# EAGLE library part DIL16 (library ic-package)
Dual In Line / Socket
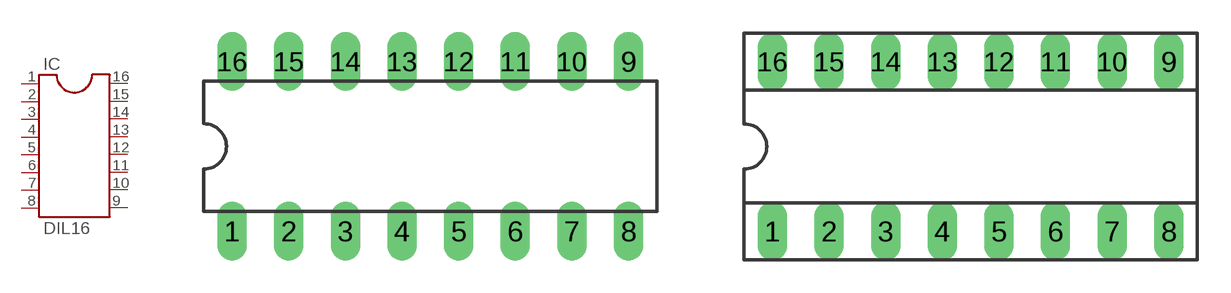
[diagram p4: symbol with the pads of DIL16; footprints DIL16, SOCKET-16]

Designator prefix IC

## DIL16  [DIL16]
1  1  pas
2  2  pas
3  3  pas
4  4  pas
5  5  pas
6  6  pas
7  7  pas
8  8  pas
9  9  pas
10  10  pas
11  11  pas
12  12  pas
13  13  pas
14  14  pas
15  15  pas
16  16  pas

## DIL16S  [SOCKET-16]
Pads as for DIL16

## Footprint DIL16 (pad centres in mm)
Dual In Line Package
drill 0.813 long: 1 -8.89,-3.81; 2 -6.35,-3.81; 3 -3.81,-3.81; 4 -1.27,-3.81; 5 1.27,-3.81; 6 3.81,-3.81; 7 6.35,-3.81; 8 8.89,-3.81; 9 8.89,3.81; 10 6.35,3.81; 11 3.81,3.81; 12 1.27,3.81; 13 -1.27,3.81; 14 -3.81,3.81; 15 -6.35,3.81; 16 -8.89,3.81

## Footprint SOCKET-16 (pad centres in mm)
Dual In Line Socket
drill 0.813 long: 1 -8.89,-3.81; 2 -6.35,-3.81; 3 -3.81,-3.81; 4 -1.27,-3.81; 5 1.27,-3.81; 6 3.81,-3.81; 7 6.35,-3.81; 8 8.89,-3.81; 9 8.89,3.81; 10 6.35,3.81; 11 3.81,3.81; 12 1.27,3.81; 13 -1.27,3.81; 14 -3.81,3.81; 15 -6.35,3.81; 16 -8.89,3.81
